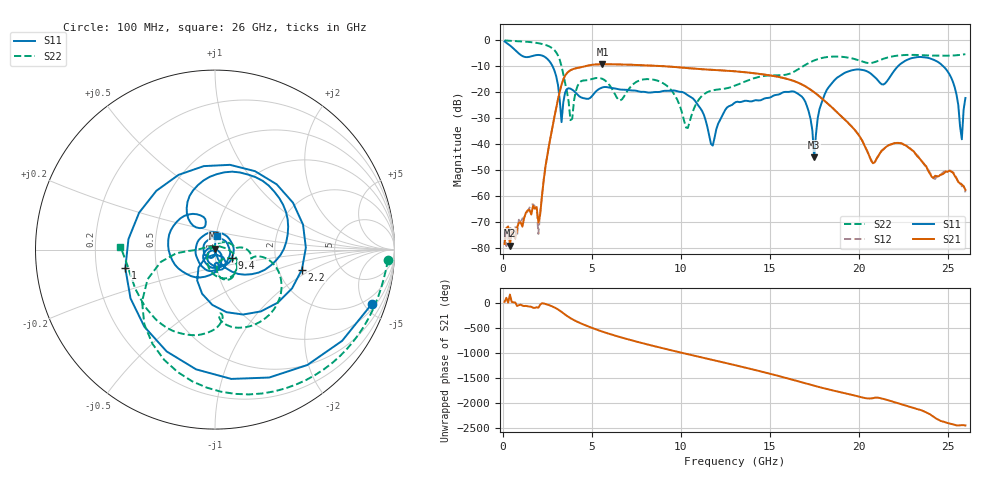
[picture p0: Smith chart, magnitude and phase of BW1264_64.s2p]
!Keysight Technologies,N5245B,MY57181159,A.13.60.06
!Date: Friday, December 18, 2020 23:55:23
!Correction: S11(Full 2 Port(1,2))
!S21(Full 2 Port(1,2))
!S12(Full 2 Port(1,2))
!S22(Full 2 Port(1,2))
!S2P File: Measurements: S11, S21, S12, S22:
# Hz S  dB  R 50
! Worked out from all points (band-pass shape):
!   260 points, 100 MHz to 26 GHz, reference 50 ohm
!   highest |S21| = -9.43 dB at 5.6 GHz (marker M1); lowest = -78.9 dB at 400 MHz (marker M2)
!   |S21| within 3 dB of the highest: 3.665 GHz to 13.53 GHz (9.868 GHz wide, 115 % of centre)
!   lowest |S11| = -45.1 dB at 17.5 GHz (marker M3), VSWR 1.01, Z = 50 + j0.557 ohm
!   |S11| at or under -10 dB: 2.782 GHz to 22.24 GHz (19.46 GHz wide, 156 % of centre); 24.73 GHz to end of sweep
!   |S22| runs from -33.8 to -0.3 dB; largest |S21 - S12| = 0.00054
!   S11 on the Smith chart (normalised r, x): 100 MHz: 1.34, -5.59; 1 GHz: 0.33, -0.09; 2.2 GHz: 2.71, -0.80; 9.4 GHz: 1.20, -0.11; 26 GHz: 1.01, +0.15
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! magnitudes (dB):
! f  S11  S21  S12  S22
! 100 MHz  -0.7  -78.3  -73.7  -0.3
! 400 MHz  -2.2  -78.9  -72.2  -0.4
! 1 GHz  -5.8  -70.0  -70.3  -0.6
! 2 GHz  -5.9  -70.0  -74.4  -1.4
! 2.2 GHz  -6.1  -59.9  -60.0  -1.6
! 3.3 GHz  -31.6  -17.2  -17.2  -10.2
! 3.8 GHz  -18.8  -11.7  -11.7  -30.8
! 4.5 GHz  -22.4  -10.4  -10.4  -15.7
! 5.6 GHz  -18.3  -9.4  -9.4  -15.0
! 8.8 GHz  -20.0  -10.1  -10.1  -16.0
! 9.4 GHz  -19.6  -10.3  -10.3  -18.8
! 10.4 GHz  -21.3  -10.9  -10.9  -33.8
! 11.8 GHz  -40.6  -11.6  -11.6  -19.4
! 13.1 GHz  -23.9  -12.2  -12.2  -17.5
! 16.4 GHz  -20.0  -15.9  -15.9  -12.2
! 17.4 GHz  -34.9  -19.6  -19.6  -8.3
! 17.5 GHz  -45.1  -20.2  -20.2  -8.0
! 18.7 GHz  -15.1  -27.3  -27.3  -6.5
! 21.7 GHz  -14.9  -40.4  -40.4  -6.7
! 24.6 GHz  -9.2  -51.7  -52.0  -6.2
! 25.8 GHz  -38.2  -55.5  -56.2  -5.8
! 26 GHz  -22.3  -57.5  -58.5  -5.6
